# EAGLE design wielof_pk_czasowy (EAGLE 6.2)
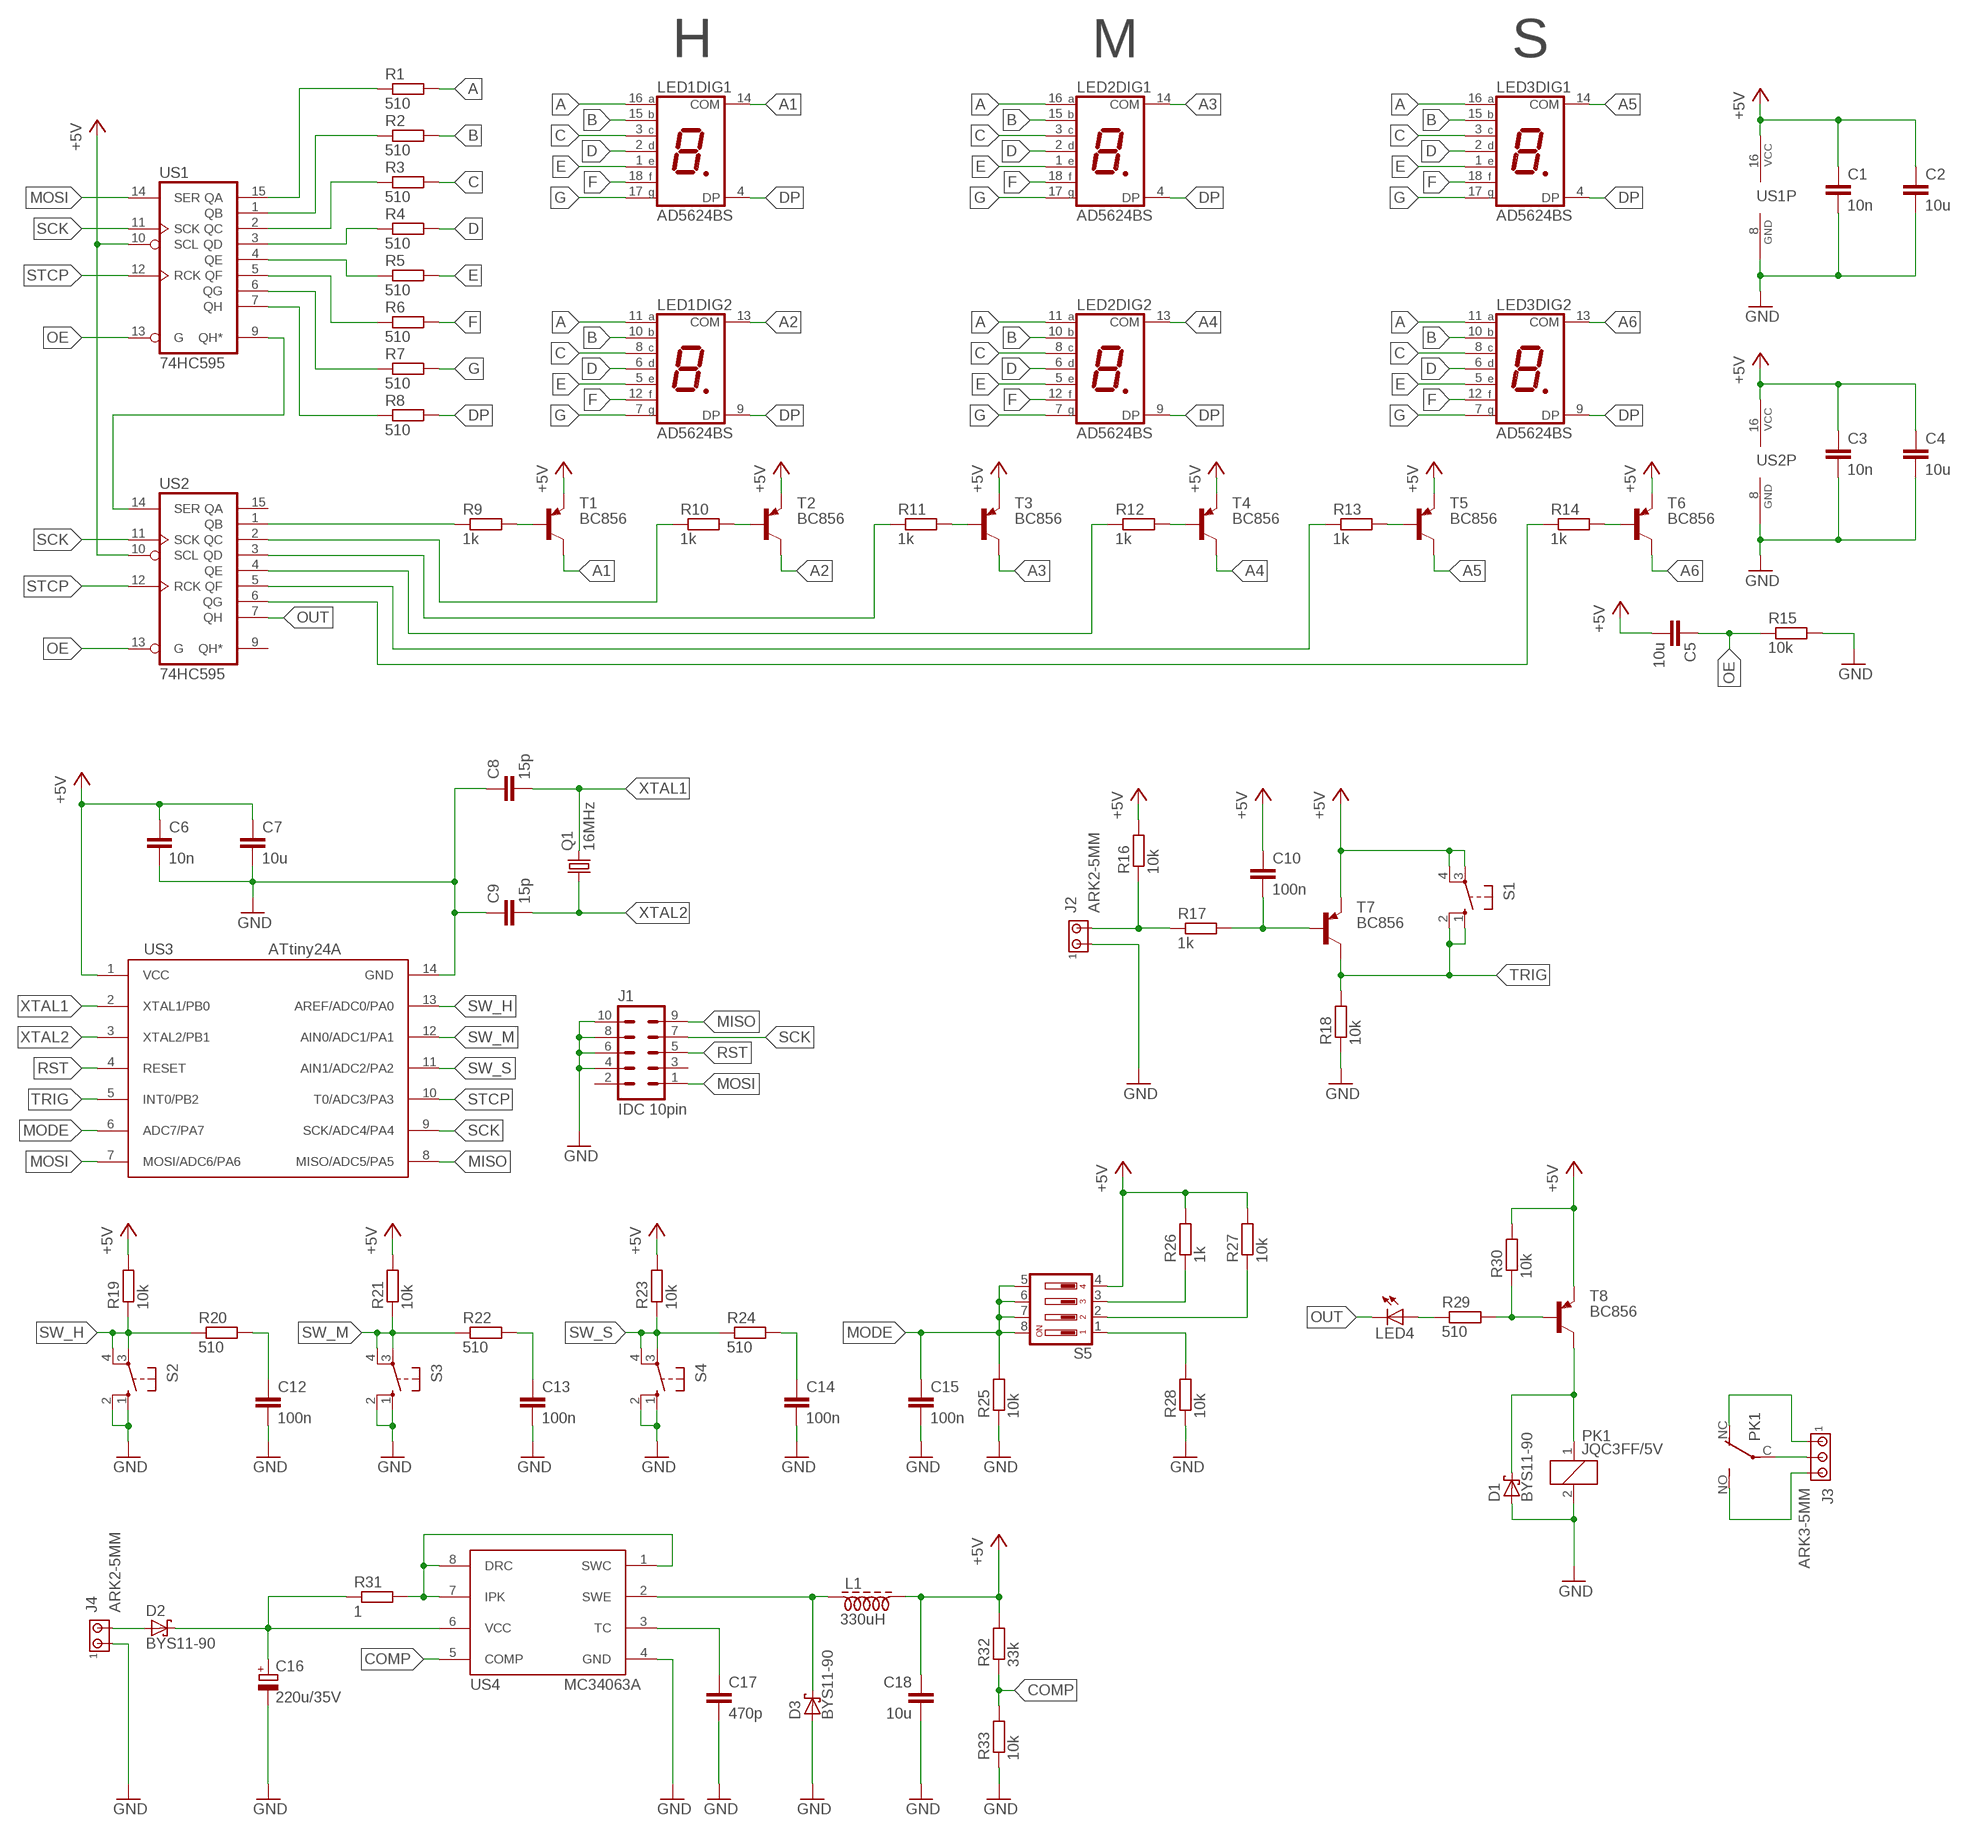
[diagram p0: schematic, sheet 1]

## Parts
C1  10n  C-EUC0805  [C0805]
C2  10u  C-EUC0805  [C0805]
C3  10n  C-EUC0805  [C0805]
C4  10u  C-EUC0805  [C0805]
C5  10u  C-EUC0805  [C0805]
C6  10n  C-EUC0805  [C0805]
C7  10u  C-EUC0805  [C0805]
C8  15p  C-EUC0805  [C0805]
C9  15p  C-EUC0805  [C0805]
C10  100n  C-EUC0805  [C0805]
C12  100n  C-EUC0805  [C0805]
C13  100n  C-EUC0805  [C0805]
C14  100n  C-EUC0805  [C0805]
C15  100n  C-EUC0805  [C0805]
C16  220u/35V  CPOL-EUE3.5-8  [E3,5-8]
C17  470p  C-EUC0805  [C0805]
C18  10u  C-EUC0805  [C0805]
D1  BYS11-90  SCHOTTKY-DIODESMD  [SMB]
D2  BYS11-90  SCHOTTKY-DIODESMD  [SMB]
D3  BYS11-90  SCHOTTKY-DIODESMD  [SMB]
J1  IDC 10pin  ML10  [ML10]
J2  ARK2-5MM  [2PIN-5MM]
J3  ARK3-5MM  [3PIN-5MM]
J4  ARK2-5MM  [2PIN-5MM]
L1  330uH  DLAWIK-PION  [L_PION]
LED1  AD5624BS  DA56-11SRWA  [DA56]
LED2  AD5624BS  DA56-11SRWA  [DA56]
LED3  AD5624BS  DA56-11SRWA  [DA56]
LED4  LED5MM  [LED5MM]
PK1  JQC3FF/5V  PK_POJED-JQC-3FG  [PK_POJED_JQC-3FG]
Q1  16MHz  CRYSTALHC49UP  [HC49UP]
R1  510  R-EU_M0805  [M0805]
R2  510  R-EU_M0805  [M0805]
R3  510  R-EU_M0805  [M0805]
R4  510  R-EU_M0805  [M0805]
R5  510  R-EU_M0805  [M0805]
R6  510  R-EU_M0805  [M0805]
R7  510  R-EU_M0805  [M0805]
R8  510  R-EU_M0805  [M0805]
R9  1k  R-EU_M0805  [M0805]
R10  1k  R-EU_M0805  [M0805]
R11  1k  R-EU_M0805  [M0805]
R12  1k  R-EU_M0805  [M0805]
R13  1k  R-EU_M0805  [M0805]
R14  1k  R-EU_M0805  [M0805]
R15  10k  R-EU_M0805  [M0805]
R16  10k  R-EU_M0805  [M0805]
R17  1k  R-EU_M0805  [M0805]
R18  10k  R-EU_M0805  [M0805]
R19  10k  R-EU_M0805  [M0805]
R20  510  R-EU_M0805  [M0805]
R21  10k  R-EU_M0805  [M0805]
R22  510  R-EU_M0805  [M0805]
R23  10k  R-EU_M0805  [M0805]
R24  510  R-EU_M0805  [M0805]
R25  10k  R-EU_M0805  [M0805]
R26  1k  R-EU_M0805  [M0805]
R27  10k  R-EU_M0805  [M0805]
R28  10k  R-EU_M0805  [M0805]
R29  510  R-EU_M0805  [M0805]
R30  10k  R-EU_M0805  [M0805]
R31  1  R-EU_M0805  [M0805]
R32  33k  R-EU_M0805  [M0805]
R33  10k  R-EU_M0805  [M0805]
S1  10-XX  [B3F-10XX]
S2  10-XX  [B3F-10XX]
S3  10-XX  [B3F-10XX]
S4  10-XX  [B3F-10XX]
S5  DS04  [DS-04]
T1  BC856  BC856ALT1SMD  [SOT23-BEC]
T2  BC856  BC856ALT1SMD  [SOT23-BEC]
T3  BC856  BC856ALT1SMD  [SOT23-BEC]
T4  BC856  BC856ALT1SMD  [SOT23-BEC]
T5  BC856  BC856ALT1SMD  [SOT23-BEC]
T6  BC856  BC856ALT1SMD  [SOT23-BEC]
T7  BC856  BC856ALT1SMD  [SOT23-BEC]
T8  BC856  BC856ALT1SMD  [SOT23-BEC]
US1  74HC595  74LS595D  [SO16]
US2  74HC595  74LS595D  [SO16]
US3  ATtiny24A  ATTINY24/44/84-SSU  [SOIC14]
US4  MC34063A  MC34063-SO8  [SO08]

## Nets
+5V: C1.1 C2.1 C3.1 C4.1 C5.2 C6.1 C7.1 C10.1 C18.1 L1.P$2 R16.2 R19.2 R21.2 R23.2 R26.2 R27.2 R30.2 R32.2 S1.3(P) S1.4(P1) S5.4 T1.E T2.E T3.E T4.E T5.E T6.E T7.E T8.E US1.10(SCL) US1.16(VCC) US2.10(SCL) US2.16(VCC) US3.1(VCC)
A: LED1.11(DIG2:A) LED1.16(DIG1:A) LED2.11(DIG2:A) LED2.16(DIG1:A) LED3.11(DIG2:A) LED3.16(DIG1:A) R1.2
A1: LED1.14(DIG1:COM) T1.C
A2: LED1.13(DIG2:COM) T2.C
A3: LED2.14(DIG1:COM) T3.C
A4: LED2.13(DIG2:COM) T4.C
A5: LED3.14(DIG1:COM) T5.C
A6: LED3.13(DIG2:COM) T6.C
B: LED1.10(DIG2:B) LED1.15(DIG1:B) LED2.10(DIG2:B) LED2.15(DIG1:B) LED3.10(DIG2:B) LED3.15(DIG1:B) R2.2
C: LED1.3(DIG1:C) LED1.8(DIG2:C) LED2.3(DIG1:C) LED2.8(DIG2:C) LED3.3(DIG1:C) LED3.8(DIG2:C) R3.2
COMP: R32.1 R33.2 US4.5(COMP)
D: LED1.2(DIG1:D) LED1.6(DIG2:D) LED2.2(DIG1:D) LED2.6(DIG2:D) LED3.2(DIG1:D) LED3.6(DIG2:D) R4.2
DP: LED1.4(DIG1:DP) LED1.9(DIG2:DP) LED2.4(DIG1:DP) LED2.9(DIG2:DP) LED3.4(DIG1:DP) LED3.9(DIG2:DP) R8.2
E: LED1.1(DIG1:E) LED1.5(DIG2:E) LED2.1(DIG1:E) LED2.5(DIG2:E) LED3.1(DIG1:E) LED3.5(DIG2:E) R5.2
F: LED1.12(DIG2:F) LED1.18(DIG1:F) LED2.12(DIG2:F) LED2.18(DIG1:F) LED3.12(DIG2:F) LED3.18(DIG1:F) R6.2
G: LED1.7(DIG2:G) LED1.17(DIG1:G) LED2.7(DIG2:G) LED2.17(DIG1:G) LED3.7(DIG2:G) LED3.17(DIG1:G) R7.2
GND: C1.2 C2.2 C3.2 C4.2 C6.2 C7.2 C8.1 C9.1 C12.2 C13.2 C14.2 C15.2 C16.- C17.2 C18.2 D1.A D3.A J1.4 J1.6 J1.8 J1.10 J2.P$1 J4.P$1 PK1.2 R15.2 R18.1 R25.1 R28.1 R33.1 S2.1(S) S2.2(S1) S3.1(S) S3.2(S1) S4.1(S) S4.2(S1) US1.8(GND) US2.8(GND) US3.14(GND) US4.4(GND)
MISO: J1.9 US3.8(MISO/ADC5/PA5)
MODE: C15.1 R25.2 S5.5 S5.6 S5.7 S5.8 US3.6(ADC7/PA7)
MOSI: J1.1 US1.14(SER) US3.7(MOSI/ADC6/PA6)
N$1: R1.1 US1.15(QA)
N$2: R2.1 US1.1(QB)
N$3: R3.1 US1.2(QC)
N$4: R4.1 US1.3(QD)
N$5: R5.1 US1.4(QE)
N$6: R6.1 US1.5(QF)
N$7: R7.1 US1.6(QG)
N$8: R8.1 US1.7(QH)
N$9: US1.9(QH*) US2.14(SER)
N$10: R9.2 T1.B
N$11: J2.P$2 R16.1 R17.1
N$12: R10.2 T2.B
N$13: R11.2 T3.B
N$14: R12.2 T4.B
N$15: R13.2 T5.B
N$16: R14.2 T6.B
N$17: R9.1 US2.1(QB)
N$18: R10.1 US2.2(QC)
N$19: R11.1 US2.3(QD)
N$20: R12.1 US2.4(QE)
N$21: R13.1 US2.5(QF)
N$22: R14.1 US2.6(QG)
N$23: C10.2 R17.2 T7.B
N$24: R27.1 S5.2
N$25: R28.2 S5.1
N$26: C12.1 R20.2
N$27: C13.1 R22.2
N$28: C14.1 R24.2
N$29: R26.1 S5.3
N$30: R29.2 R30.1 T8.B
N$31: D2.A J4.P$2
N$32: C16.+ D2.C R31.1 US4.6(VCC)
N$33: LED4.A R29.1
N$34: J3.P$2 PK1.C(COM)
N$35: J3.P$1 PK1.NC
N$36: J3.P$3 PK1.NO
N$37: R31.2 US4.1(SWC) US4.7(IPK) US4.8(DRC)
N$38: C17.1 US4.3(TC)
N$39: D3.C L1.P$1 US4.2(SWE)
N$40: D1.C PK1.1 T8.C
OE: C5.1 R15.1 US1.13(G) US2.13(G)
OUT: LED4.K(C) US2.7(QH)
RST: J1.5 US3.4(RESET)
SCK: J1.7 US1.11(SCK) US2.11(SCK) US3.9(SCK/ADC4/PA4)
STCP: US1.12(RCK) US2.12(RCK) US3.10(T0/ADC3/PA3)
SW_H: R19.1 R20.1 S2.3(P) S2.4(P1) US3.13(AREF/ADC0/PA0)
SW_M: R21.1 R22.1 S3.3(P) S3.4(P1) US3.12(AIN0/ADC1/PA1)
SW_S: R23.1 R24.1 S4.3(P) S4.4(P1) US3.11(AIN1/ADC2/PA2)
TRIG: R18.2 S1.1(S) S1.2(S1) T7.C US3.5(INT0/PB2)
XTAL1: C8.2 Q1.2 US3.2(XTAL1/PB0)
XTAL2: C9.2 Q1.1 US3.3(XTAL2/PB1)
Unconnected: J1.2 J1.3 US2.9(QH*) US2.15(QA)

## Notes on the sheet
- H | M | S

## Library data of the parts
C1-C10 C12-C15 C17 C18 = rcl:C-EU: CAPACITOR, European symbol
C16 = rcl:CPOL-EU: POLARIZED CAPACITOR, European symbol
D1-D3 = diode:SCHOTTKY-DIODE: Schottky Diode
J1 = con-harting-ml:ML10: HARTING; OC_FARNELL: unknown; OC_NEWARK: unknown
J2 J4 = zlacza_futrzak:ARK2: ARK 2
J3 = zlacza_futrzak:ARK3: ARK 3 Raster 5mm i 3,5mm
L1 = inne_futrzak:DLAWIK
LED1-LED3 = display-kingbright:DA56-11: 14.22mm (0.56INCH) DUAL DIGIT NUMERIC DISPLAYS Source: www.kingbright.com .. DA56-11SRWA.pdf; OC_FARNELL: unknown; OC_NEWARK: unknown
LED4 = led:LED: LED
PK1 = inne_futrzak:PK_POJED
Q1 = crystal:CRYSTAL: CRYSTAL; OC_FARNELL: unknown; OC_NEWARK: unknown
R1-R33 = rcl:R-EU_: RESISTOR, European symbol
S1-S4 = switch-omron:10-XX: OMRON SWITCH; MPN: B3F-1000; OC_FARNELL: 176432; OC_NEWARK: 36M3542
S5 = switch-dil:DS04: DIL/CODE SWITCH; OC_FARNELL: 9471570; OC_NEWARK: unknown
T1-T8 = transistor-pnp:BC856*: PNP Transistror
US1 US2 = scalaki_futrzak:74*595: 8-bit SHIFT REGISTER, output latch
US3 = scalaki_futrzak:ATTINY24/44/84
US4 = scalaki_futrzak:MC34063

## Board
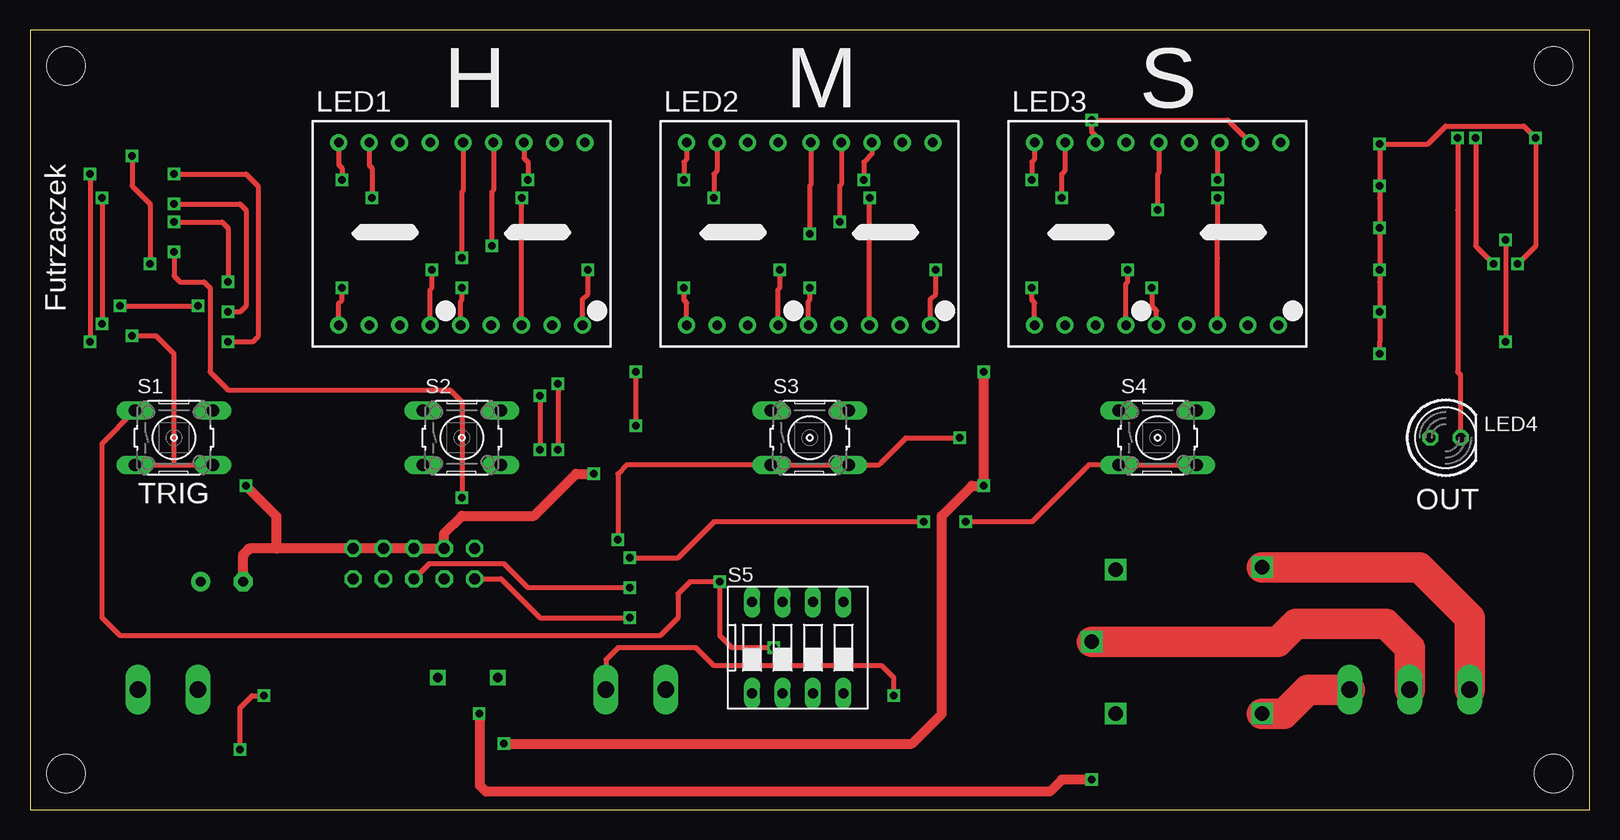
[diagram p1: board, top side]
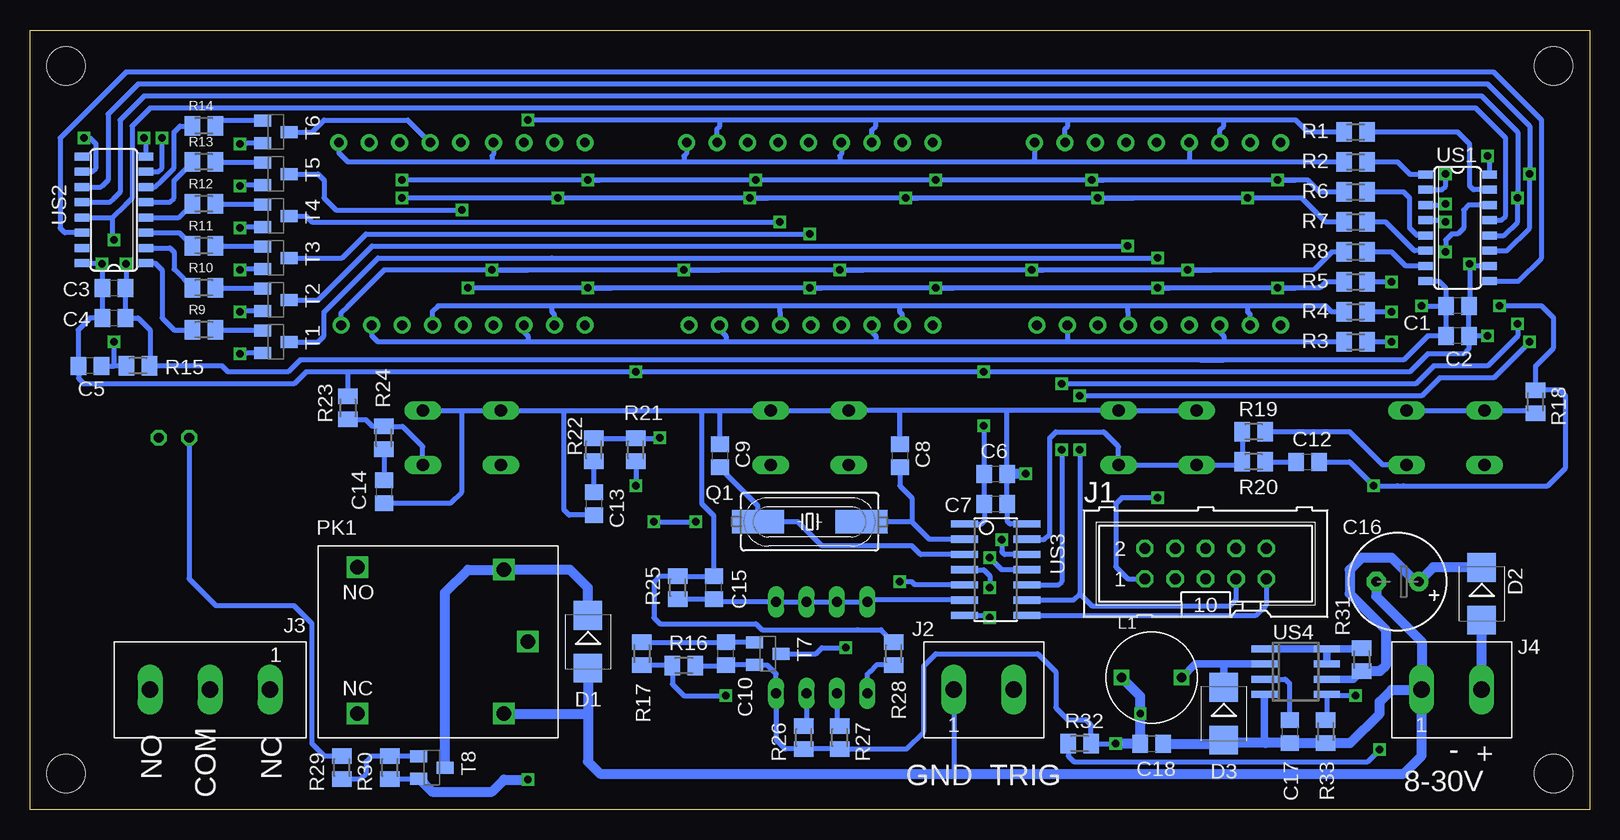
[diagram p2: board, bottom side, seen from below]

Size 130 x 65 mm. Coordinates in mm from the lower left corner, seen from the top.
Outline: 0,0 130,0 130,65 0,65 0,0
Copper layers (1*16): Top 0.035mm / dielectric 1.5mm / Bottom 0.035mm
Design rules: minimum track width 10mil, minimum drill 23mil, track to track 8mil, track to pad 8mil, pad to pad 8mil, via to via 8mil, smd to smd 8mil, copper to edge 40mil, drill to drill 8mil, minimum pad ring 10mil, minimum via ring 8mil, stop-mask expansion 4mil, vias tented up to drill 0mil, thermal gap 10mil
Holes 3.2 mm at 3,62 127,62 3,3 127,3

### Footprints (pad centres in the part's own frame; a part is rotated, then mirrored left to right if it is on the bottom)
C0805 = smd 1.3 x 1.5: 1 -0.95,0; 2 0.95,0
E3,5-8 = drill 0.813 pad 1.6: + -1.778,0 | drill 0.813 pad 1.6 octagon: - 1.778,0
SMB = smd 2.4 x 2.4: A 2.2,0; C -2.2,0
ML10 = drill 0.914 octagon: 1 -5.08,-1.27; 2 -5.08,1.27; 3 -2.54,-1.27; 4 -2.54,1.27; 5 0,-1.27; 6 0,1.27; 7 2.54,-1.27; 8 2.54,1.27; 9 5.08,-1.27; 10 5.08,1.27
2PIN-5MM = drill 1.4 long: P$1 -2.5,0; P$2 2.5,0
3PIN-5MM = drill 1.4 long: P$1 -5,0; P$2 0,0; P$3 5,0
L_PION = drill 0.8 square: P$1 -2.5,0; P$2 2.5,0
DA56 = drill 0.8 pad 1.422: 1 -10.26,-7.62; 2 -7.72,-7.62; 3 -5.18,-7.62; 4 -2.64,-7.62; 5 -0.1,-7.62; 6 2.44,-7.62; 7 4.98,-7.62; 8 7.52,-7.62; 9 10.06,-7.62; 10 10.26,7.62; 11 7.72,7.62; 12 5.18,7.62; 13 2.64,7.62; 14 0.1,7.62; 15 -2.64,7.62; 16 -5.18,7.62; 17 -7.72,7.62; 18 -10.26,7.62
LED5MM = drill 0.813 octagon: A -1.27,0; K 1.27,0
PK_POJED_JQC-3FG = drill 1.2 square: 1 5.5,6; 2 5.5,-6; C 7.5,0; NC -6.7,-6; NO -6.7,6.2
HC49UP = smd 4.318 x 1.93: 1 -4.318,0; 2 4.318,0
M0805 = smd 1.3 x 1.6: 1 -0.95,0; 2 0.95,0
B3F-10XX = drill 1.016 long: 1 -3.251,2.261; 2 3.251,2.261; 3 -3.251,-2.261; 4 3.251,-2.261
DS-04 = drill 0.813 long: 1 -3.81,-3.81; 2 -1.27,-3.81; 3 1.27,-3.81; 4 3.81,-3.81; 5 3.81,3.81; 6 1.27,3.81; 7 -1.27,3.81; 8 -3.81,3.81
SOT23-BEC = smd 1 x 1.4: B -0.95,-1.1; C 0,1.1; E 0.95,-1.1
SO16 = smd 0.66 x 1.2: 1 -4.445,-2.673; 2 -3.175,-2.673; 3 -1.905,-2.673; 4 -0.635,-2.673; 5 0.635,-2.673; 6 1.905,-2.673; 7 3.175,-2.673; 8 4.445,-2.673; 9 4.445,2.673; 10 3.175,2.673; 11 1.905,2.673; 12 0.635,2.673; 13 -0.635,2.673; 14 -1.905,2.673; 15 -3.175,2.673; 16 -4.445,2.673
SOIC14 = smd 0.61 x 2.21: 1 -3.81,-2.603; 2 -2.54,-2.603; 3 -1.27,-2.603; 4 0,-2.603; 5 1.27,-2.603; 6 2.54,-2.603; 7 3.81,-2.603; 8 3.81,2.603; 9 2.54,2.603; 10 1.27,2.603; 11 0,2.603; 12 -1.27,2.603; 13 -2.54,2.603; 14 -3.81,2.603
SO08 = smd 0.6 x 2.2: 1 -1.905,-2.6; 2 -0.635,-2.6; 3 0.635,-2.6; 4 1.905,-2.6; 5 1.905,2.6; 6 0.635,2.6; 7 -0.635,2.6; 8 -1.905,2.6

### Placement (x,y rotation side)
C1  11,42 180 bottom
C2  11,39.5 180 bottom
C3  123,43.5 0 bottom
C4  123,41 0 bottom
C5  125,37 180 bottom
C6  49.5,28 0 bottom
C7  49.5,25.5 0 bottom
C8  57.5,29.5 270 bottom
C9  72.5,29.5 270 bottom
C10  72,13 90 bottom
C12  23.5,29 0 bottom
C13  83,25.5 270 bottom
C14  100.5,26.5 270 bottom
C15  73,18.5 90 bottom
C16  16,19 180 bottom
C17  25,6.5 270 bottom
C18  36.5,5.5 0 bottom
D1  83.5,14 270 bottom
D2  9,18 270 bottom
D3  30.5,8 270 bottom
J1  32,20.5 0 bottom
J2  50.5,10 0 bottom
J3  115,10 180 bottom
J4  11.5,10 0 bottom
L1  36.5,11 180 bottom
LED1  36,48 0 top
LED2  65,48 0 top
LED3  94,48 0 top
LED4  118,31 0 top
PK1  96,14 0 bottom
Q1  65,24 0 bottom
R1  19.5,56.5 180 bottom
R2  19.5,54 180 bottom
R3  19.5,39 180 bottom
R4  19.5,41.5 180 bottom
R5  19.5,44 180 bottom
R6  19.5,51.5 180 bottom
R7  19.5,49 180 bottom
R8  19.5,46.5 180 bottom
R9  115.5,40 0 bottom
R10  115.5,43.5 0 bottom
R11  115.5,47 0 bottom
R12  115.5,50.5 0 bottom
R13  115.5,54 0 bottom
R14  115.5,57 0 bottom
R15  121,37 0 bottom
R16  75.5,12 0 bottom
R17  79,13 90 bottom
R18  4.5,34 270 bottom
R19  28,31.5 0 bottom
R20  28,29 0 bottom
R21  79.5,30 270 bottom
R22  83,30 270 bottom
R23  103.5,33.5 90 bottom
R24  100.5,31 270 bottom
R25  76,18.5 270 bottom
R26  65.5,6 270 bottom
R27  62.5,6 270 bottom
R28  58,13 270 bottom
R29  104,3.5 270 bottom
R30  100,3.5 270 bottom
R31  19,12.5 90 bottom
R32  42.5,5.5 0 bottom
R33  22,6.5 90 bottom
S1  12,31 0 top
S2  36,31 0 top
S3  65,31 0 top
S4  94,31 0 top
S5  64,13.5 0 top
T1  109.5,39 270 bottom
T2  109.5,42.5 270 bottom
T3  109.5,46 270 bottom
T4  109.5,49.5 270 bottom
T5  109.5,53 270 bottom
T6  109.5,56.5 270 bottom
T7  68.5,13 270 bottom
T8  96.5,3.5 270 bottom
US1  11,48.5 270 bottom
US2  123,50 90 bottom
US3  49.5,20 270 bottom
US4  24.5,11.5 270 bottom

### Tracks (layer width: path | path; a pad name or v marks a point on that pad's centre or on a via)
+5V  (via drill 0.6)
  Top 0.406: v112.5,38 112.5,39 112.5,41 v112.5,41.5 112.5,44 v112.5,45 112.5,48 v112.5,48.5 112.5,51 v112.5,52 v112.5,55.5 116.5,55.5 118,57 124.5,57 v125.5,56 125.5,47 v124,45.5 | v8.5,54.5 8.5,52 10,50.5 v10,45.5 | v50.5,32 v50.5,36.5 | S1.3 12,28.74 | 12,28.74 12,38 10.5,39.5 v8.5,39.5 | 12,28.74 S1.4
  Top 0.813: v39.5,5.5 73.5,5.5 76,8 76,24.5 78.5,27 v79.5,27 v79.5,36.5 | v88.5,2.5 86,2.5 85,1.5 38,1.5 37.5,2 37.5,7.95 v37.45,8
  Bottom 0.406: T6.E 111.95,55.55 v112.5,55.5 | T1.E 111.95,38.05 v112.5,38 | T5.E 112.45,52.05 v112.5,52 | T4.E 112.45,48.55 v112.5,48.5 | T3.E 112.45,45.05 v112.5,45 | T2.E 112.45,41.55 v112.5,41.5 | US2.10 124.83,53.17 124.5,53.5 124.5,55.5 125,56 v125.5,56 | US2.16 124.06,45.55 v124,45.5 124,43.55 C3.1 C4.1 125,41 126,40 126,37.05 C5.2 125.95,35.95 125.5,35.5 108,35.5 107,36.5 103.5,36.5 | C2.1 C1.1 10,42.05 v10,45.5 9.82,45.33 US1.10 | US1.16 8.33,54.33 v8.5,54.5 | C2.1 10.05,38.45 10.5,38 13.5,38 15,36.5 v50.5,36.5 v79.5,36.5 103.5,36.5 | US3.1 50.69,23.81 50.45,24.05 C7.1 C6.1 50.45,31.95 v50.5,32 | R30.2 T8.E | v8.5,39.5 C2.1 | v39.5,5.5 R32.2 41.55,7.05 42,7.5 43.5,7.5 44.5,8.5 44.5,11.5 46,13 54.5,13 55.5,12 55.5,6.5 56.95,5.05 R27.2 R26.2 67.05,5.05 67.81,5.81 S5.4 67.81,11.31 68.55,12.05 T7.E C10.1 72.05,12 R16.2 | S1.4 17.24,28.74 20,31.5 R19.2 | R21.2 v79.5,27 | R23.2 103.5,36.5
  Bottom 0.813: T8.E 97.1,2.1 96.5,1.5 91.5,1.5 90.5,2.5 v88.5,2.5 | L1.P$2 37.45,9.45 v37.45,8 C18.1 v39.5,5.5
A  (via drill 0.6)
  Top 0.406: LED3.11 99.84,57.5 v88.5,57.5 88.5,56.5 88.82,56.18 LED3.16
  Bottom 0.406: R1.2 23.5,56.5 24.5,57.5 30.5,57.5 | 30.5,57.5 43.5,57.5 | 43.5,57.5 59.5,57.5 | 59.5,57.5 72.5,57.5 | 72.5,57.5 v88.5,57.5 | LED2.11 72.72,56.78 72.5,57 72.5,57.5 | LED2.16 59.82,56.68 59.5,57 59.5,57.5 | LED1.11 43.72,56.78 43.5,57 43.5,57.5 | LED1.16 30.82,56.68 30.5,57 30.5,57.5
A1  (via drill 0.6)
  Top 0.406: v36,46 36,51.5 36.1,51.6 LED1.14
  Bottom 0.406: T1.C 106,39 105.5,39.5 105.5,41.5 101,46 86.5,46 v36,46
A2  (via drill 0.6)
  Top 0.406: v38.5,47 38.5,51.5 38.64,51.64 LED1.13
  Bottom 0.406: T2.C 106,42.5 101.5,47 v38.5,47
A3  (via drill 0.6)
  Top 0.406: v65,48 65,52 65.1,52.1 LED2.14
  Bottom 0.406: T3.C 104,46 102,48 v65,48
A4  (via drill 0.6)
  Top 0.406: v67.5,49 67.5,52 67.64,52.14 LED2.13
  Bottom 0.406: T4.C 107,49.5 106.5,49 v67.5,49
A5  (via drill 0.6)
  Top 0.406: v94,50 94,53 94.1,53.1 LED3.14
  Bottom 0.406: T5.C 106,53 105.5,52.5 105.5,51 104.5,50 v94,50
A6
  Bottom 0.406: T6.C 106.5,56.5 105.5,57.5 98.52,57.5 LED3.13
B
  Bottom 0.406: R2.2 33.5,54 | 33.5,54 46.5,54 | 46.5,54 62.5,54 | 62.5,54 75.5,54 | 75.5,54 91.5,54 | 91.5,54 103.5,54 104,54.5 104.26,54.76 LED3.10 | LED1.15 33.36,54.14 33.5,54 | LED1.10 46.26,54.24 46.5,54 | LED3.15 91.36,54.64 91.5,54.5 91.5,54 | LED2.10 75.26,54.74 75.5,54.5 75.5,54 | LED2.15 62.36,54.64 62.5,54.5 62.5,54
C
  Bottom 0.406: R3.2 30.5,39 | 30.5,39 43.5,39 | 43.5,39 59.5,39 | 59.5,39 72,39 | 72,39 88.5,39 | 88.5,39 101,39 101.5,39.5 101.5,40.36 LED3.8 | LED3.3 88.82,39.82 88.5,39.5 88.5,39 | LED2.8 72.52,40.02 72,39.5 72,39 | LED2.3 59.82,39.82 59.5,39.5 59.5,39 | LED1.3 30.82,39.82 30.5,39.5 30.5,39 | LED1.8 43.52,39.02 43.5,39
COMP  (via drill 0.6)
  Top 0.406: v17.5,5 17.5,8.5 18.5,9.5 v19.5,9.5
  Bottom 0.406: R33.2 21.9,7.55 US4.5 21.8,9.5 v19.5,9.5 | R32.1 43.45,4.45 43,4 18.5,4 v17.5,5
D
  Bottom 0.406: R4.2 21.5,41.5 22,42 28.5,42 | 28.5,42 38.5,42 | 38.5,42 57.5,42 | 57.5,42 67.5,42 | 67.5,42 86.5,42 | 86.5,42 96,42 96.44,41.56 LED3.6 | LED1.2 28.28,41.28 28.5,41.5 28.5,42 | LED1.6 38.44,41.44 38.5,41.5 38.5,42 | LED2.2 57.28,41.28 57.5,41.5 57.5,42 | LED2.6 67.44,41.44 67.5,41.5 67.5,42 | LED3.2 86.28,41.28 86.5,41.5 86.5,42
DP  (via drill 0.6)
  Top 0.406: LED1.4 33.36,43.36 33.5,43.5 v33.5,45 | LED1.9 46.06,42.56 46.5,43 v46.5,45 | LED2.4 62.36,43.36 62.5,43.5 v62.5,45 | LED2.9 75.06,42.56 75.5,43 v75.5,45 | LED3.4 91.36,43.86 91.5,44 v91.5,45
  Bottom 0.406: R8.2 21.5,46.5 23,45 31.5,45 | 31.5,45 v33.5,45 | v33.5,45 45.5,45 | 45.5,45 v46.5,45 | v46.5,45 60.5,45 | 60.5,45 v62.5,45 | v62.5,45 72.5,45 | 72.5,45 v75.5,45 | v75.5,45 88.5,45 | 88.5,45 v91.5,45 | v91.5,45 100.5,45 103.5,42 104.06,41.44 LED3.9 | v33.5,45 31.5,45 | v46.5,45 45.5,45 | v62.5,45 60.5,45 | v75.5,45 72.5,45 | v91.5,45 88.5,45
E  (via drill 0.6)
  Top 0.406: v93.5,43.5 93.5,42 93.9,41.6 LED3.5 | LED1.1 25.74,42.24 26,42.5 v26,43.5 | LED1.5 35.9,42.4 36,42.5 v36,43.5 | LED2.1 54.74,42.26 54.5,42.5 v54.5,43.5 | LED2.5 64.9,42.4 65,42.5 v65,43.5 | LED3.1 83.74,42.26 83.5,42.5 v83.5,43.5
  Bottom 0.406: R5.2 22,44 22.5,43.5 24.5,43.5 | 24.5,43.5 v26,43.5 | v26,43.5 35,43.5 | 35,43.5 v36,43.5 | v36,43.5 53,43.5 | 53,43.5 v54.5,43.5 | v54.5,43.5 64,43.5 | 64,43.5 v65,43.5 | v65,43.5 81.5,43.5 | 81.5,43.5 v83.5,43.5 | v83.5,43.5 v93.5,43.5 | v26,43.5 24.5,43.5 | v36,43.5 35,43.5 | v54.5,43.5 53,43.5 | v65,43.5 64,43.5 | v83.5,43.5 81.5,43.5
F  (via drill 0.6)
  Top 0.406: v99,52.5 99,55.44 LED3.12 | LED3.18 83.74,54.24 83.5,54 v83.5,52.5 | LED2.12 70.18,54.68 69.5,54 v69.5,52.5 | LED2.18 54.74,54.24 54.5,54 v54.5,52.5 | LED1.12 41.18,54.32 41.5,54 v41.5,52.5 | LED1.18 25.74,53.76 26,53.5 v26,52.5
  Bottom 0.406: R6.2 22.5,51.5 23.5,52.5 24.5,52.5 | 24.5,52.5 v26,52.5 | v26,52.5 40.5,52.5 | 40.5,52.5 v41.5,52.5 | v41.5,52.5 54,52.5 | 54,52.5 v54.5,52.5 | v54.5,52.5 v69.5,52.5 | v69.5,52.5 70,52.5 | 70,52.5 82.5,52.5 | 82.5,52.5 v83.5,52.5 | v83.5,52.5 v99,52.5 | v83.5,52.5 82.5,52.5 | v69.5,52.5 70,52.5 | v54.5,52.5 54,52.5 | v41.5,52.5 40.5,52.5 | v26,52.5 24.5,52.5
G  (via drill 0.6)
  Top 0.406: v86,51 86,53 86.28,53.28 LED3.17 | LED2.17 57.28,53.28 57,53 v57,51 | LED1.17 28.28,53.72 28.5,53.5 v28.5,51 | LED3.7 98.98,45.98 v99,51 | LED2.7 69.98,50.98 v70,51 | LED1.7 40.98,50.98 v41,51
  Bottom 0.406: R7.2 22,49 24,51 v28.5,51 | v28.5,51 29.5,51 | 29.5,51 38,51 | 38,51 v41,51 | v41,51 56,51 | 56,51 v57,51 | v57,51 68.5,51 | 68.5,51 v70,51 | v70,51 85.5,51 | 85.5,51 v86,51 | v57,51 56,51 | v28.5,51 29.5,51 | 85.5,51 98,51 v99,51 | v70,51 68.5,51 | v41,51 38,51
GND  (via drill 0.6)
  Top 0.406: v120.5,56 120.5,47 v122,45.5 | v7.5,42 v14,42
  Top 0.813: 20.55,21.77 J1.10 J1.8 J1.6 J1.4 34.54,23.04 36,24.5 42,24.5 45.5,28 v47,28 | 20.55,21.77 20.55,24.45 v18,27 | 20.55,21.77 18.27,21.77 18,21.5 17.78,21.28 C16.-
  Bottom 0.406: US2.8 120.33,55.83 v120.5,56 | v122,45.5 122,43.55 C3.2 C4.2 121,41 120,40 120,37.05 R15.2 114,37 113.5,36.5 108.5,36.5 107.5,37.5 32.5,37.5 | C1.2 C2.2 13.5,39.5 15.5,37.5 30.5,37.5 | US1.8 12.55,44.05 12,43.5 12,42.05 C1.2 | 30.5,37.5 32.5,37.5 | US3.14 48.31,23.81 48.5,24 48.55,24.05 C7.2 48.55,27.5 C6.2 48.55,33.21 48.5,33.26 | 32.5,37.5 30.5,37.5 | 48.5,33.26 S2.2 S2.1 | 48.5,33.26 57.5,33.26 | 57.5,33.26 S3.1 S3.2 72.5,33.26 | 85.5,33.26 S4.1 94,33.26 | 85.5,33.26 76,33.26 74,33.26 | 74,33.26 72.5,33.26 | S4.2 94,33.26 | C9.1 72.5,33.26 | C8.1 57.5,33.26 | J2.P$1 53,3 | v7.5,42 4,42 3,41 3,38.5 4.5,37 R18.1 4.45,35 2.5,35 2,34.5 2,28.5 3.5,27 15.5,27 | v14,42 C1.2 | C12.2 20,29 18.5,27.5 v18,27 | v18,27 16,27 | 16,27 15.5,27 | v18,27 16,27 | 16,27 15.5,27 | C13.2 85.05,24.55 85.5,25 85.5,33.26 | C14.2 94.95,25.55 94,26.5 94,33.26 | 74,33.26 74,25.5 73,24.5 C15.2 R25.1 77.55,19.45 78,19 78,16 77.5,15.5 69.5,15.5 69,15 61,15 59.05,15 R28.1 | v18,27 16,27
  Bottom 0.61: US4.4 27.1,5.65 27,5.55
  Bottom 0.813: C16.- 17.78,17.78 14,14 J4.P$1 | D1.A 83.5,8 | 83.5,8 83.5,4 82.5,3 53,3 15.5,3 14,4.5 J4.P$1 | PK1.2 83.5,8 | C18.2 30.8,5.5 D3.A 30.25,5.55 27,5.55 C17.2 R33.1 19.95,5.55 17.5,8 17.5,9 16.5,10 J4.P$1 | v47,28 48.05,28 48.55,27.5
MISO
  Bottom 0.406: US3.8 27.81,16.19 27,17 26.92,17.08 J1.9
MODE
  Bottom 0.406: R25.2 C15.1 72.76,17.31 S5.5 S5.6 S5.7 S5.8 60.04,17.46 US3.6
MOSI  (via drill 0.6)
  Top 0.406: J1.1 39.27,19.23 41,17.5 41.5,17 42,16.5 42.5,16 v50,16 | v12,46.5 12,44.5 12.5,44 14.5,44 15,43.5 15,36.5 16.5,35 35,35 36,34 v36,26
  Bottom 0.406: US1.14 10.1,50.41 10.5,50 10.5,48.5 11,48 11.5,48 12,47.5 v12,46.5 | US3.7 50.19,16.19 v50,16 | v36,26 39,26 39.5,25.5 39.5,20.23 38.5,19.23 J1.1
N$1
  Bottom 0.406: US1.15 9.68,51.67 10,52 10,55.5 11,56.5 R1.1
N$2
  Bottom 0.406: US1.1 14.95,52.95 16,54 R2.1
N$3  (via drill 0.6)
  Top 0.406: v12,53 18,53 19,52 19,39.45 R3.1 v16.5,39
  Bottom 0.406: US1.2 12.32,51.67 12,52 v12,53 | v16.5,39 R3.1
N$4  (via drill 0.6)
  Top 0.406: v12,50.5 17.5,50.5 18,50 18,42 17.5,41.5 v16.5,41.5
  Bottom 0.406: US1.3 12.1,50.41 v12,50.5 | v16.5,41.5 R4.1
N$5  (via drill 0.6)
  Top 0.406: v12,49 16,49 16.5,48.5 v16.5,44
  Bottom 0.406: US1.4 12.13,49.13 v12,49 | v16.5,44 R5.1
N$6
  Bottom 0.406: US1.5 14.37,47.87 15,48.5 15,51 15.5,51.5 R6.1
N$7
  Bottom 0.406: US1.6 14.6,46.59 17,49 R7.1
N$8
  Bottom 0.406: US1.7 15.32,45.33 16.5,46.5 R8.1
N$9
  Bottom 0.406: US1.9 5.95,44.05 4,46 4,57.5 8,61.5 122,61.5 127.5,56 127.5,48.5 127.09,48.09 US2.14
N$10
  Bottom 0.406: T1.B 114.5,39.95 R9.2
N$11  (via drill 0.6)
  Top 0.406: v72,9.5 72,11 71,12 57,12 55.5,13.5 49,13.5 48,12.5 J2.P$2
  Bottom 0.406: R17.1 76.5,12.05 R16.1 76.45,10.45 75.5,9.5 v72,9.5
N$12
  Bottom 0.406: T2.B 114.5,43.45 R10.2
N$13
  Bottom 0.406: T3.B 114.5,46.95 R11.2
N$14
  Bottom 0.406: T4.B 114.5,50.45 R12.2
N$15
  Bottom 0.406: T5.B 114.5,53.95 R13.2
N$16
  Bottom 0.406: T6.B 114.5,57.45 R14.2
N$17
  Bottom 0.406: US2.1 119.56,45.55 119,45 119,41 118,40 R9.1
N$18
  Bottom 0.406: US2.2 118.33,46.83 118,46.5 118,45.05 R10.1
N$19
  Bottom 0.406: US2.3 117.55,48.09 R11.1
N$20
  Bottom 0.406: US2.4 117.58,49.37 R12.1
N$21
  Bottom 0.406: US2.5 118.36,50.63 118,51 118,52.45 R13.1
N$22
  Bottom 0.406: US2.6 119.59,51.91 119,52.5 118,53.5 118,55.5 118,56.5 117.5,57 R14.1
N$23
  Bottom 0.406: T7.B C10.2 R17.2
N$24
  Bottom 0.406: S5.2 62.73,6.68 R27.1
N$25
  Bottom 0.406: R28.2 59.45,12.05 60,11.5 60.19,11.31 S5.1
N$26
  Bottom 0.406: R20.2 C12.1
N$27
  Bottom 0.406: C13.1 R22.2
N$28
  Bottom 0.406: R24.2 C14.1
N$29
  Bottom 0.406: S5.3 65.27,6.68 R26.1
N$30
  Bottom 0.406: T8.B R30.1 101.55,4.45 102,4 102,3 102.45,2.55 R29.2
N$31
  Bottom 0.813: J4.P$2 D2.A
N$32
  Bottom 0.61: US4.6 19.68,10.87 R31.1
  Bottom 0.813: D2.C 13.02,20.2 C16.+ 14.5,19 16,20.5 16.5,21 19,21 20,20 20,18 17,15 17,12 17.45,11.55 R31.1
N$33
  Bottom 0.406: R29.1 105.45,4.45 106.5,5.5 106.5,15.5 108,17 114.5,17 115.5,18 116.73,19.23 LED4.A
N$34
  Top 2.54: PK1.C 104,14 105.5,15.5 113,15.5 115,13.5 J3.P$2
N$35
  Top 2.54: PK1.NC 104.5,8 106.5,10 J3.P$1
N$36
  Top 2.54: PK1.NO 115.8,20.2 120,16 J3.P$3
N$37
  Bottom 0.61: US4.7 US4.8 | US4.1 US4.8 | US4.8 19.05,13.4 R31.2
N$38
  Bottom 0.406: C17.1 25,10.5 25.36,10.87 US4.3
N$39
  Bottom 0.61: US4.2 30.5,12.13 | 30.5,12.13 32.87,12.13 L1.P$1 | D3.C 30.5,12.13
N$40
  Bottom 0.813: D1.C 83.5,18.5 85,20 PK1.1 93.5,20 95.4,18.1 T8.C
OE  (via drill 0.6)
  Top 0.406: v123,47.5 v123,39
  Bottom 0.406: US1.13 7.37,49.13 7,49.5 7,56 9,58 9.5,58.5 120,58.5 121.5,57 121.5,51 122,50.5 123.14,49.37 | US2.13 123.14,49.37 | 123.14,49.37 123.14,47.63 v123,47.5 | R15.1 123,37 | 123,37 v123,39 | C5.1 123,37
OUT  (via drill 0.6)
  Top 0.406: v119,56 119,50 119,36.5 119.27,36.23 LED4.K
  Bottom 0.406: US2.7 119.33,53.17 119,53.5 v119,56
RST  (via drill 0.6)
  Top 0.406: v50,18.5 41.5,18.5 39.5,20.5 33.27,20.5 J1.5
  Bottom 0.406: US3.4 50.5,20 50,19.5 v50,18.5
SCK  (via drill 0.6)
  Top 0.406: v5,53 v5,39 | v42.5,34.5 v42.5,30
  Bottom 0.406: US1.11 6.91,46.59 5,48.5 v5,53 5,57 8.5,60.5 121,60.5 123.5,58 123.5,52.5 124,52 124.09,51.91 US2.11 | US3.9 45.46,17.46 45,17.46 43.04,17.46 42.5,18 | v5,39 8,36 12.5,36 14,34.5 v42.5,34.5 | v42.5,30 42.5,18 | 42.5,18 41.5,17 30,17 29.5,17.5 29.46,17.54 J1.7
STCP  (via drill 0.6)
  Top 0.406: v6,51 v6,40.5 | v44,35.5 v44,30
  Bottom 0.406: US1.12 7.13,47.87 6,49 v6,51 6,56.5 9,59.5 120.5,59.5 121,59 122.5,57.5 122.5,51.5 123,51 123.36,50.63 US2.12 | v6,40.5 6,39.5 8.5,37 13,37 14.5,35.5 v44,35.5 | v44,30 44,19 44.27,18.73 US3.10
SW_H
  Bottom 0.406: R19.1 R20.1 29.21,28.74 S2.3 S2.4 39.25,30.25 39.5,30.5 40.5,31.5 44.5,31.5 45,31 45,23 45.46,22.54 US3.13
SW_M  (via drill 0.6)
  Top 0.406: v49,22.5 49,28 49.74,28.74 S3.3 S3.4 70.74,28.74 71,29 73,31 v77.5,31
  Bottom 0.406: v49,22.5 49,22 49,21.5 48.77,21.27 US3.12 | R22.1 R21.1 77.55,30.95 v77.5,31
SW_S  (via drill 0.6)
  Top 0.406: v50,21 54,21 57,24 v74.5,24 | S4.4 S4.3 88.24,28.74 88,28.5 83.5,24 v78,24
  Bottom 0.406: US3.11 49,20 v50,21 | S4.4 97.25,30.25 97.5,30.5 98.95,31.95 R24.1 101.45,31.95 102,32.5 103.45,32.5 R23.1 | v78,24 v74.5,24
TRIG  (via drill 0.6)
  Top 0.406: v62,13.5 58.5,13.5 57.5,14.5 v57.5,19 55,19 54,18 54,16 52.5,14.5 7.5,14.5 6.5,15.5 6,16 6,30.51 S1.1
  Bottom 0.406: S1.2 S1.1 5.29,33.26 R18.2 | T7.C 64.5,13 64,13.5 v62,13.5 | US3.5 55.73,18.73 56.23,18.73 56.5,19 v57.5,19
XTAL1
  Bottom 0.406: US3.2 55.04,22.54 56.5,24 | 56.5,24 Q1.2 | C8.2 57.5,27 56.5,26 56.5,24
XTAL2
  Bottom 0.406: US3.3 55.77,21.27 56.5,22 64,22 66,24 Q1.1 69.32,25.32 69.5,25.5 72.5,28.5 C9.2

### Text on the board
tPlace: H | M | S | Futrzaczek | TRIG | OUT
bPlace: + - | 8-30V | GND TRIG | NC | NO | COM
